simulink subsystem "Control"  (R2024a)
settings: Solver=VariableStepAuto  StartTime=0.0  StopTime=10.0  RelTol=1e-3
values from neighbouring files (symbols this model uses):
  Control = ControlType.Simple    [TotemPole_PFCData.m]
  Tsc_fast = 1e-5    (= 1e-05)    [TotemPole_PFCData.m]
  Tsc_slow = 0.01    [TotemPole_PFCData.m]
undefined symbols (not defined in the file or in its folder): I
libraries: simulink x10, simulink_extras x2, slpidlib x2, dspsigops x1

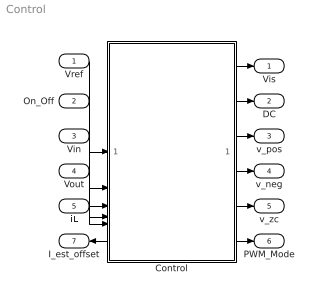
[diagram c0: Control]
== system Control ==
  Vref : Inport
  On_Off : Inport  Port=2
  Vin : Inport  Port=3
  Vout : Inport  Port=4
  iL : Inport  Port=5
  Control : Subsystem  Variant=on  VariantControl=Control
  Vis : Outport
  DC : Outport  Port=2
  v_pos : Outport  Port=3
  v_neg : Outport  Port=4
  v_zc : Outport  Port=5
  PWM_Mode : Outport  Port=6
  I_est_offset : Outport  Port=7
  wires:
  On_Off/1 -> Control/2(On_Off)
  iL/1 -> Control/5(iL)
  Control/6(PWM_Mode) -> PWM_Mode/1
  Vin/1 -> Control/3(Vin)
  Vout/1 -> Control/4(Vout)
  Control/1(Vis) -> Vis/1
  Control/2(DC) -> DC/1
  Control/3(v_pos) -> v_pos/1
  Control/4(v_neg) -> v_neg/1
  Control/5(v_zc) -> v_zc/1
  Control/7(I_est_offset) -> I_est_offset/1
  Vref/1 -> Control/1(Vref)

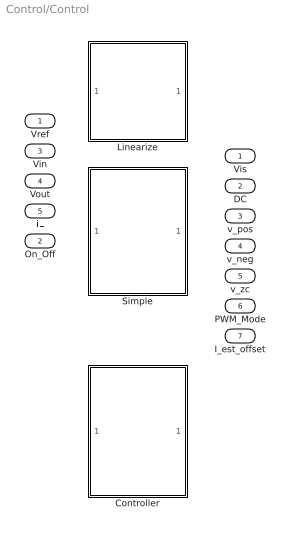
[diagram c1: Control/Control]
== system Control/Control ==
  Vref : Inport
  On_Off : Inport  Port=2
  Vin : Inport  Port=3
  Vout : Inport  Port=4
  iL : Inport  Port=5
  Controller : Subsystem  VariantControl=Control == ControlType.Detailed
  Linearize : Subsystem  VariantControl=Control == ControlType.Linearization
  Simple : Subsystem  VariantControl=Control == ControlType.Simple
  Vis : Outport
  DC : Outport  Port=2
  v_pos : Outport  Port=3
  v_neg : Outport  Port=4
  v_zc : Outport  Port=5
  PWM_Mode : Outport  Port=6
  I_est_offset : Outport  Port=7

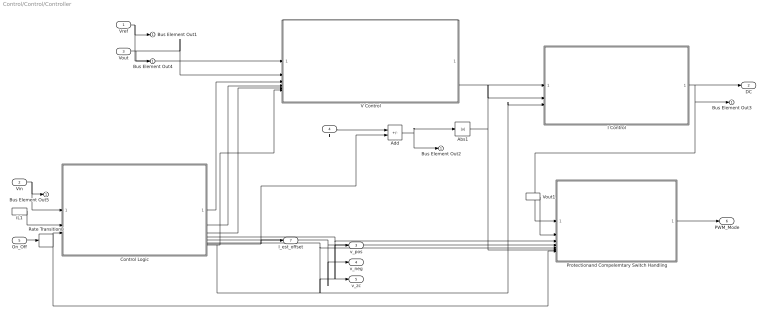
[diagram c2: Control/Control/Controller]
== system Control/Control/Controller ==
  Vref : Inport
  Vin : Inport  Port=2
  Vout : Inport  Port=3
  iL : Inport  Port=4
  On_Off : Inport  Port=5
  Abs1 : Abs
  Add : Sum  Inputs=+-
  Control Logic : Subsystem
  I Control : ModelReference  ModelNameDialog=I_Control  ModelReferenceVersion=9.283  CopyOfModelProtected=on
  Protectionand Compelemtary Switch Handling : Subsystem
  Rate Transition8 : RateTransition  OutPortSampleTime=1/100e3
  V Control : Subsystem
  Vout1 : InportShadow  Port=3
  iL1 : InportShadow  Port=4
  Bus Element Out{1..5} (5 alike) : Outport
  DC : Outport  Port=2
  v_pos : Outport  Port=3
  v_neg : Outport  Port=4
  v_zc : Outport  Port=5
  PWM_Mode : Outport  Port=6
  I_est_offset : Outport  Port=7
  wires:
  Add/1 -> Abs1/1, Bus Element Out2/1
  iL/1 -> Add/1
  Vref/1 -> Bus Element Out1/1, V Control/1(Vref)
  I Control/1 -> Protectionand Compelemtary Switch Handling/1(DC), Bus Element Out3/1, DC/1
  V Control/1(I_slowref) -> I Control/1
  Vin/1 -> Bus Element Out5/1, Control Logic/1(Vin)
  iL1/1 -> Control Logic/2(Iin)
  On_Off/1 -> Rate Transition8/1
  Control Logic/1(Vin_scaled) -> V Control/3(Vin_scaled)
  Control Logic/2(redge) -> V Control/4(redge)
  Control Logic/3(fedge) -> V Control/5(fedge)
  Control Logic/7(I_est_offset) -> I_est_offset/1, Add/2
  Vout/1 -> Bus Element Out4/1, V Control/2(Vout)
  Control Logic/6(V_zc) -> v_zc/1, Protectionand Compelemtary Switch Handling/5(vin_zc)
  Control Logic/4(V_pos) -> Protectionand Compelemtary Switch Handling/3(vin_p), v_pos/1
  Control Logic/5(V_neg) -> v_neg/1, Protectionand Compelemtary Switch Handling/4(vin_n)
  Abs1/1 -> Protectionand Compelemtary Switch Handling/6(I_abs), I Control/2
  Protectionand Compelemtary Switch Handling/1(PWM_Mode) -> PWM_Mode/1
  Vout1/1 -> Protectionand Compelemtary Switch Handling/2(Vout)
  Control Logic/8(EN_ALIGN) -> I Control/3, V Control/6(On_Off1)
  Rate Transition8/1 -> Protectionand Compelemtary Switch Handling/7(On_off_1), Control Logic/3(EN_M)

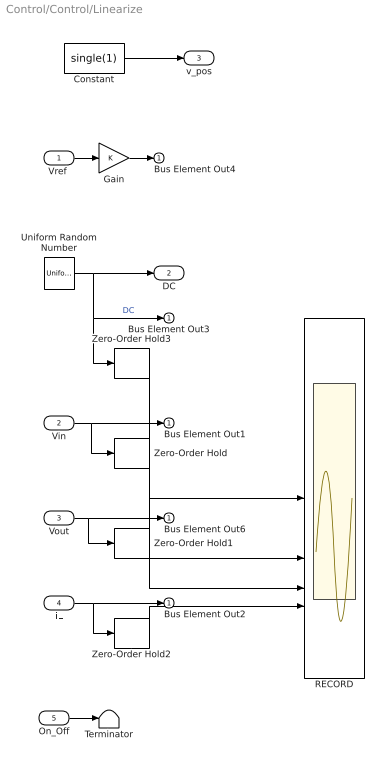
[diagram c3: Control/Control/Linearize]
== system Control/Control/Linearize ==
  "Vref " : Inport
  Vin : Inport  Port=2
  Vout : Inport  Port=3
  iL : Inport  Port=4
  On_Off : Inport  Port=5
  Constant : Constant  Value=single(1)
  Gain : Gain
  RECORD : Scope  NumInputPorts=4
  Terminator : Terminator
  Uniform Random Number : UniformRandomNumber  Minimum=-0.1  Maximum=0.1  SampleTime=Tsc_fast
  Zero-Order Hold{,1..3} (4 alike) : ZeroOrderHold  SampleTime=Tsc_fast
  Bus Element Out{1..4,6} (5 alike) : Outport
  DC : Outport  Port=2
  v_pos : Outport  Port=3
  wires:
  iL/1 -> Zero-Order Hold2/1, Bus Element Out2/1
  Vout/1 -> Zero-Order Hold1/1, Bus Element Out6/1
  Vin/1 -> Zero-Order Hold/1, Bus Element Out1/1
  Uniform Random Number/1 -> Bus Element Out3/1, Zero-Order Hold3/1, DC/1  "DC"
  Constant/1 -> v_pos/1
  Zero-Order Hold3/1 -> RECORD/1
  Zero-Order Hold/1 -> RECORD/2
  Zero-Order Hold1/1 -> RECORD/3
  Zero-Order Hold2/1 -> RECORD/4
  "Vref "/1 -> Gain/1
  Gain/1 -> Bus Element Out4/1
  On_Off/1 -> Terminator/1

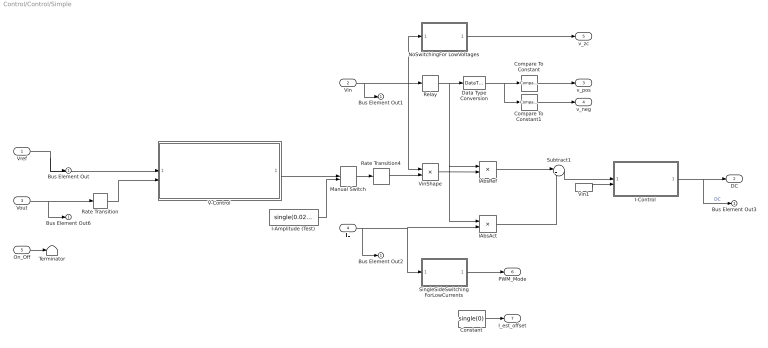
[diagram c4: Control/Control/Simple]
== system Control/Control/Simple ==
  Vref : Inport
  Vin : Inport  Port=2
  Vout : Inport  Port=3
  iL : Inport  Port=4
  On_Off : Inport  Port=5
  Compare To Constant : simulink/Logic and Bit Operations/Compare To Constant  relop===  const=1  OutDataTypeStr=boolean
  Compare To Constant1 : simulink/Logic and Bit Operations/Compare To Constant  relop===  const=-1  OutDataTypeStr=boolean
  Constant : Constant  Value=single(0)  SampleTime=Tsc_fast
  Data Type Conversion : DataTypeConversion  OutDataTypeStr=int8
  I-Amplitude (Test) : Constant  Value=single(0.025*10)  SampleTime=Tsc_fast
  I-Control : Subsystem  Variant=on  VariantControl=I-Control
  IAbsAct : Product
  IAbsRef : Product
  Manual Switch : ManualSwitch
  NoSwitchingFor LowVoltages : Subsystem  mask{vTh=2, perc=4}
      mask prompts: vTh "Voltage Threshold [V]"; perc "Hysteresis [+/- %]"
  Rate Transition : RateTransition  OutPortSampleTime=Tsc_slow
  Rate Transition4 : RateTransition  Deterministic=off  OutPortSampleTime=Tsc_fast
  Relay : Relay  OnSwitchValue=0.08  OffSwitchValue=-0.08  OffOutputValue=-1  ZeroCross=off
  SingleSideSwitching ForLowCurrents : Subsystem  mask{iTh=2, hyst=0.1}
      mask prompts: iTh "Current Threshold [A]"; hyst "Hysteresis [+/- A]"
  Subtract1 : Sum  Inputs=|+-
  Terminator : Terminator
  V-Control : Subsystem
  Vin1 : InportShadow  Port=2
  VinShape : Product
  Bus Element Out{,1..3,6} (5 alike) : Outport
  DC : Outport  Port=2
  v_pos : Outport  Port=3
  v_neg : Outport  Port=4
  v_zc : Outport  Port=5
  PWM_Mode : Outport  Port=6
  I_est_offset : Outport  Port=7
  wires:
  Rate Transition/1 -> V-Control/2(V_out)
  I-Control/1(DC) -> DC/1, Bus Element Out3/1  "DC"
  Vin1/1 -> I-Control/2(Vin)
  IAbsRef/1 -> Subtract1/1
  IAbsAct/1 -> Subtract1/2
  Constant/1 -> I_est_offset/1
  Vin/1 -> Relay/1, NoSwitchingFor LowVoltages/1(v), VinShape/1, Bus Element Out1/1
  VinShape/1 -> IAbsRef/2
  Rate Transition4/1 -> VinShape/2
  Vout/1 -> Rate Transition/1, Bus Element Out6/1
  I-Amplitude (Test)/1 -> Manual Switch/2
  Vref/1 -> Bus Element Out/1, V-Control/1(V_ref)
  SingleSideSwitching ForLowCurrents/1(PWM_Mode) -> PWM_Mode/1
  NoSwitchingFor LowVoltages/1(v_zc) -> v_zc/1
  Relay/1 -> Data Type Conversion/1, IAbsAct/1, IAbsRef/1
  Data Type Conversion/1 -> Compare To Constant1/1, Compare To Constant/1
  Subtract1/1 -> I-Control/1(delta_I)
  V-Control/1("I_ref ") -> Manual Switch/1
  Manual Switch/1 -> Rate Transition4/1
  iL/1 -> IAbsAct/2, SingleSideSwitching ForLowCurrents/1(i), Bus Element Out2/1
  On_Off/1 -> Terminator/1
  Compare To Constant/1 -> v_pos/1
  Compare To Constant1/1 -> v_neg/1

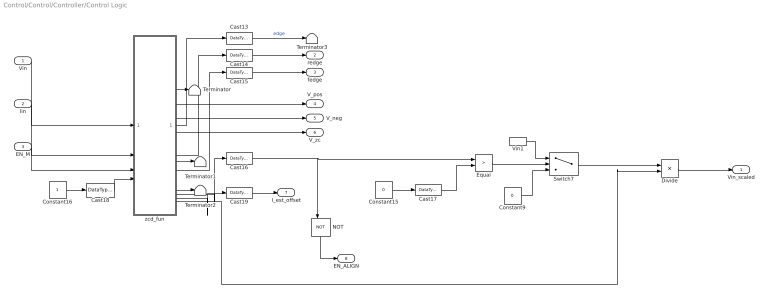
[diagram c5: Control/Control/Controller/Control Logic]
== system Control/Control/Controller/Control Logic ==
  Vin : Inport
  Iin : Inport  Port=2
  EN_M : Inport  Port=3
  Cast{13..17} (5 alike) : DataTypeConversion  OutDataTypeStr=boolean
  Cast18 : DataTypeConversion  OutDataTypeStr=single
  Cast19 : DataTypeConversion  OutDataTypeStr=single
  Constant15 : Constant  Value=0  OutDataTypeStr=single
  Constant16 : Constant
  Constant9 : Constant  Value=0  OutDataTypeStr=single
  Divide : Product  Inputs=**
  Equal : RelationalOperator  Operator=>  OutDataTypeStr=boolean  RndMeth=Simplest
  NOT : Logic  Operator=NOT  IconShape=distinctive  AllPortsSameDT=off  OutDataTypeStr=boolean
  Switch7 : Switch  Criteria=u2 > Threshold
  Terminator{,1..3} (4 alike) : Terminator
  Vin1 : InportShadow
  zcd_fun : MATLAB Function  TreatAsAtomicUnit=on
  Vin_scaled : Outport
  redge : Outport  Port=2
  fedge : Outport  Port=3
  V_pos : Outport  Port=4
  V_neg : Outport  Port=5
  V_zc : Outport  Port=6
  I_est_offset : Outport  Port=7
  EN_ALIGN : Outport  Port=8
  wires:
  zcd_fun/12(Vrms_inv2_o) -> Divide/2
  EN_M/1 -> zcd_fun/3(EN_M_in)
  Cast14/1 -> redge/1
  Constant9/1 -> Switch7/3
  Cast16/1 -> Equal/1, NOT/1
  Vin1/1 -> Switch7/1
  zcd_fun/5(V_pos) -> V_pos/1
  Iin/1 -> zcd_fun/2(Iin)
  Cast18/1 -> zcd_fun/4(Vth_in)
  zcd_fun/11(cedge) -> Terminator2/1
  Vin/1 -> zcd_fun/1(Vin)
  zcd_fun/3(fedge) -> Cast15/1
  zcd_fun/1(edge) -> Cast13/1
  Constant16/1 -> Cast18/1
  Equal/1 -> Switch7/2
  zcd_fun/2(redge) -> Cast14/1
  Cast19/1 -> I_est_offset/1
  Cast15/1 -> fedge/1
  zcd_fun/8(En_pos_align) -> Cast16/1
  Switch7/1 -> Divide/1
  Constant15/1 -> Cast17/1
  zcd_fun/10(I_offset2_o) -> Cast19/1
  Cast17/1 -> Equal/2
  Cast13/1 -> Terminator3/1  "edge"
  zcd_fun/4(Vpeak_o) -> Terminator/1
  zcd_fun/9(I_offset_o) -> Terminator1/1
  zcd_fun/7(V_zc) -> V_zc/1
  zcd_fun/6(V_neg) -> V_neg/1
  Divide/1 -> Vin_scaled/1
  NOT/1 -> EN_ALIGN/1

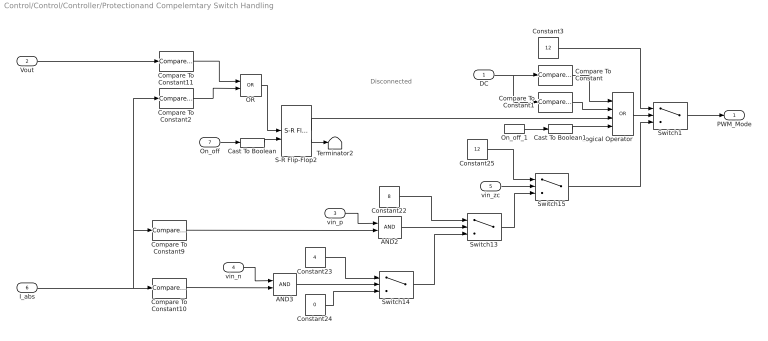
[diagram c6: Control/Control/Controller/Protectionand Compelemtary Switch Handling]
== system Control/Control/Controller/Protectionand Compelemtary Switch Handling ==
  note: Disconnected
  DC : Inport
  Vout : Inport  Port=2
  vin_p : Inport  Port=3
  vin_n : Inport  Port=4
  vin_zc : Inport  Port=5
  I_abs : Inport  Port=6
  On_off : Inport  Port=7
  AND2 : Logic  IconShape=distinctive  AllPortsSameDT=off  OutDataTypeStr=boolean
  AND3 : Logic  IconShape=distinctive  AllPortsSameDT=off  OutDataTypeStr=boolean
  Cast To Boolean : DataTypeConversion  OutDataTypeStr=boolean
  Cast To Boolean1 : DataTypeConversion  OutDataTypeStr=boolean
  Compare To Constant : simulink/Logic and Bit Operations/Compare To Constant  relop=<=  const=-0.001  OutDataTypeStr=boolean
  Compare To Constant1 : simulink/Logic and Bit Operations/Compare To Constant  relop=>=  const=1.1  OutDataTypeStr=boolean
  Compare To Constant10 : simulink/Logic and Bit Operations/Compare To Constant  relop=<  const=2  OutDataTypeStr=boolean
  Compare To Constant11 : simulink/Logic and Bit Operations/Compare To Constant  relop=>=  const=80  OutDataTypeStr=boolean
  Compare To Constant2 : simulink/Logic and Bit Operations/Compare To Constant  relop=>=  const=25  OutDataTypeStr=boolean
  Compare To Constant9 : simulink/Logic and Bit Operations/Compare To Constant  relop=<  const=2  OutDataTypeStr=boolean
  Constant22 : Constant  Value=8  OutDataTypeStr=uint16
  Constant23 : Constant  Value=4  OutDataTypeStr=uint16
  Constant24 : Constant  Value=0  OutDataTypeStr=uint16
  Constant25 : Constant  Value=12  OutDataTypeStr=uint16
  Constant3 : Constant  Value=12  OutDataTypeStr=uint16
  Logical Operator : Logic  Operator=OR  Inputs=4  AllPortsSameDT=off  OutDataTypeStr=boolean
  OR : Logic  Operator=OR  IconShape=distinctive  AllPortsSameDT=off  OutDataTypeStr=boolean
  On_off_1 : InportShadow  Port=7
  S-R Flip-Flop2 : simulink_extras/Flip Flops/S-R Flip-Flop  initial_condition=0
  Switch{1,13..15} (4 alike) : Switch  Criteria=u2 > Threshold
  Terminator2 : Terminator
  PWM_Mode : Outport
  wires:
  Compare To Constant10/1 -> AND3/2
  Switch1/1 -> PWM_Mode/1
  S-R Flip-Flop2/2 -> Terminator2/1
  Constant25/1 -> Switch15/1
  AND3/1 -> Switch14/2
  Switch15/1 -> Switch1/3
  Cast To Boolean/1 -> S-R Flip-Flop2/2
  OR/1 -> S-R Flip-Flop2/1
  Constant3/1 -> Switch1/1
  vin_zc/1 -> Switch15/2
  Constant24/1 -> Switch14/3
  Compare To Constant9/1 -> AND2/2
  vin_p/1 -> AND2/1
  Logical Operator/1 -> Switch1/2
  Compare To Constant11/1 -> OR/1
  Switch13/1 -> Switch15/3
  Compare To Constant/1 -> Logical Operator/1
  DC/1 -> Compare To Constant/1, Compare To Constant1/1
  Compare To Constant1/1 -> Logical Operator/2
  AND2/1 -> Switch13/2
  Constant22/1 -> Switch13/1
  Switch14/1 -> Switch13/3
  vin_n/1 -> AND3/1
  Vout/1 -> Compare To Constant11/1
  Constant23/1 -> Switch14/1
  On_off/1 -> Cast To Boolean/1
  I_abs/1 -> Compare To Constant2/1, Compare To Constant9/1, Compare To Constant10/1
  S-R Flip-Flop2/1 -> Logical Operator/3
  On_off_1/1 -> Cast To Boolean1/1
  Compare To Constant2/1 -> OR/2
  Cast To Boolean1/1 -> Logical Operator/4

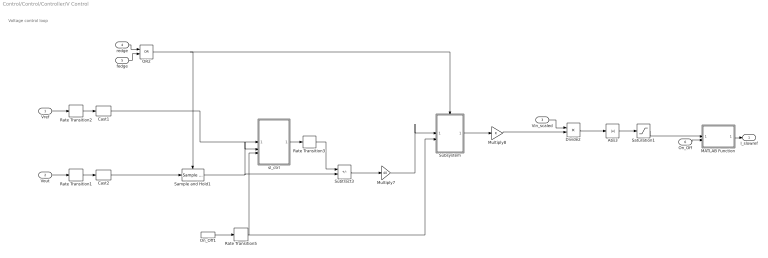
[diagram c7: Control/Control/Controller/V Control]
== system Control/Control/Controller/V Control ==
  note: Voltage control loop
  Vref : Inport
  Vout : Inport  Port=2
  Vin_scaled : Inport  Port=3
  redge : Inport  Port=4
  fedge : Inport  Port=5
  On_Off : Inport  Port=6
  Abs3 : Abs
  Cast1 : DataTypeConversion  OutDataTypeStr=single
  Cast2 : DataTypeConversion  OutDataTypeStr=single
  Divide2 : Product  Inputs=**
  MATLAB Function : MATLAB Function  TreatAsAtomicUnit=on
  Multiply7 : Gain  Gain=40
  Multiply8 : Gain
  OR2 : Logic  Operator=OR  IconShape=distinctive  AllPortsSameDT=off  OutDataTypeStr=boolean
  On_Off1 : InportShadow  Port=6
  Rate Transition1 : RateTransition  OutPortSampleTime=Tsc_fast
  Rate Transition2 : RateTransition  OutPortSampleTime=Tsc_slow
  Rate Transition3 : RateTransition  OutPortSampleTime=Tsc_slow
  Rate Transition5 : RateTransition  OutPortSampleTime=Tsc_slow
  Sample and Hold1 : dspsigops/Sample and Hold  trig=Rising edge  initCond=0  latchinput=off
  Saturation1 : Saturate  UpperLimit=30  LowerLimit=-30
  Subsystem : Subsystem
  Subtract3 : Sum  Inputs=+-
  sl_ctrl : MATLAB Function  TreatAsAtomicUnit=on
  I_slowref : Outport
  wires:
  Rate Transition5/1 -> Subsystem/2(In2), sl_ctrl/3(RST)
  Saturation1/1 -> MATLAB Function/1(I_ref)
  Rate Transition1/1 -> Cast2/1
  Rate Transition3/1 -> Subtract3/1
  OR2/1 -> Sample and Hold1/Trigger, Subsystem/Enable
  Abs3/1 -> Saturation1/1
  Cast1/1 -> sl_ctrl/1(V_ref)
  Vin_scaled/1 -> Divide2/1
  sl_ctrl/1(V_slowref) -> Rate Transition3/1
  Rate Transition2/1 -> Cast1/1
  Vout/1 -> Rate Transition1/1
  redge/1 -> OR2/1
  Subtract3/1 -> Multiply7/1
  Sample and Hold1/1 -> Subtract3/2, sl_ctrl/2(V_init)
  Multiply7/1 -> Subsystem/1(In1)
  Subsystem/1(Out1) -> Multiply8/1
  fedge/1 -> OR2/2
  Cast2/1 -> Sample and Hold1/1
  Divide2/1 -> Abs3/1
  MATLAB Function/1(I_slowref) -> I_slowref/1
  Multiply8/1 -> Divide2/2
  On_Off/1 -> MATLAB Function/2(RST)
  Vref/1 -> Rate Transition2/1
  On_Off1/1 -> Rate Transition5/1

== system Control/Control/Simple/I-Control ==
  delta_I : Inport
  Vin : Inport  Port=2
  IIR_Control : Subsystem  VariantControl=IControl == IControlType.IIR_2p2z
  PI Controller : Subsystem  VariantControl=IControl == IControlType.PI
  DC : Outport

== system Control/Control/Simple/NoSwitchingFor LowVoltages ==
  v : Inport
  Abs : Abs  ZeroCross=off
  NOT : Logic  Operator=NOT  IconShape=distinctive  AllPortsSameDT=off  OutDataTypeStr=boolean
  Relay : Relay  OnSwitchValue=vTh*(1+perc/100)  OffSwitchValue=vTh*(1-perc/100)  OutDataTypeStr=boolean  ZeroCross=off
  v_zc : Outport
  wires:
  Abs/1 -> Relay/1
  v/1 -> Abs/1
  Relay/1 -> NOT/1
  NOT/1 -> v_zc/1

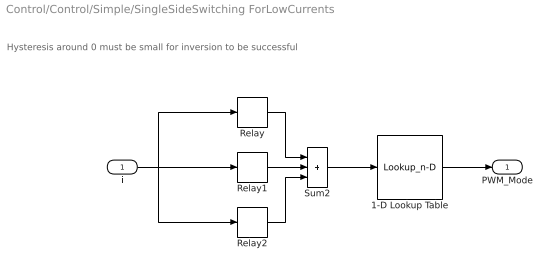
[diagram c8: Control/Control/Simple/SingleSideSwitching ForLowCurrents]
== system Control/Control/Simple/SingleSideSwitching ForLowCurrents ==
  note: Hysteresis around 0 must be small for inversion to be successful
  i : Inport
  1-D Lookup Table : Lookup_n-D  NumberOfTableDimensions=1  LookupTableObject=''  BreakpointsForDimension1=[0,1,2,3]  BreakpointsForDimension1FirstPoint=10  BreakpointsForDimension2FirstPoint=10  BreakpointsForDimension1Spacing=12  BreakpointsForDimension2Spacing=12  IndexSearchMethod=Evenly spaced points  Table=[0,4,8,0]  InterpMethod=Flat  DiagnosticForOutOfRangeInput=Error  InternalRulePriority=Speed  RndMeth=Simplest
  Relay : Relay  OnSwitchValue=iTh+hyst  OffSwitchValue=iTh-hyst  OutDataTypeStr=int8  ZeroCross=off
  Relay1 : Relay  OnSwitchValue=0.02  OffSwitchValue=-0.02  OutDataTypeStr=int8  ZeroCross=off
  Relay2 : Relay  OnSwitchValue=-iTh+hyst  OffSwitchValue=-iTh-hyst  OutDataTypeStr=int8  ZeroCross=off
  Sum2 : Sum  Inputs=+++
  PWM_Mode : Outport
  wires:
  Relay1/1 -> Sum2/2
  i/1 -> Relay2/1, Relay1/1, Relay/1
  Relay2/1 -> Sum2/3
  Relay/1 -> Sum2/1
  Sum2/1 -> 1-D Lookup Table/1
  1-D Lookup Table/1 -> PWM_Mode/1

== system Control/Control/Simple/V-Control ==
  V_ref : Inport
  V_out : Inport  Port=2
  "PI Controller no Saturation " : slpidlib/PID Controller  Controller=PI  Form=Parallel  TimeDomain=Discrete-time  UseExternalTs=off  SampleTime=Tsc_slow  IntegratorMethod=Forward Euler  FilterMethod=Forward Euler  ControllerParametersSource=internal  P=0.08  I=0.7  UseKiTs=off  D=0  UseExternalDerivativeSource=off  N=100  UseFilter=on  TunerSelectOption=Transfer Function Based (PID Tuner App)  ZeroCross=off  InitialConditionSource=internal  InitialConditionForIntegrator=0  InitialConditionForFilter=0  DifferentiatorICPrevScaledInput=0  ExternalReset=none  TrackingMode=off  Kt=1  LimitOutput=on  SatLimitsSource=internal  UpperSaturationLimit=0.5  LowerSaturationLimit=-1  LinearizeAsGain=on  AntiWindupMode=clamping  Kb=1  LimitIntegrator=off  UpperIntegratorSaturationLimit=inf  LowerIntegratorSaturationLimit=-inf  POutMin=[]  POutMax=[]  IOutMin=[]  IOutMax=[]  DOutMin=[]  DOutMax=[]  NOutMin=[]  NOutMax=[]  SumOutMin=[]  SumOutMax=[]  SaturationOutMin=[]  SaturationOutMax=[]  PParamMin=[]  PParamMax=[]  IParamMin=[]  IParamMax=[]  DParamMin=[]  DParamMax=[]  NParamMin=[]  NParamMax=[]  KbParamMin=[]  KbParamMax=[]  KtParamMin=[]  KtParamMax=[]  KbOutMin=[]  KbOutMax=[]  KtOutMin=[]  KtOutMax=[]  IntegratorOutMin=[]  IntegratorOutMax=[]  FilterOutMin=[]  FilterOutMax=[]  SumI1OutMin=[]  SumI1OutMax=[]  SumI2OutMin=[]  SumI2OutMax=[]  SumI3OutMin=[]  SumI3OutMax=[]  SumI4OutMin=[]  SumI4OutMax=[]  SumDOutMin=[]  SumDOutMax=[]  DifferentiatorOutMin=[]  DifferentiatorOutMax=[]  FilterDiffOutCoefMin=[]  FilterDiffOutCoefMax=[]  ReciprocalOutMin=[]  ReciprocalOutMax=[]  SumDenOutMin=[]  SumDenOutMax=[]  SumNumOutMin=[]  SumNumOutMax=[]  DivideOutMin=[]  DivideOutMax=[]  UdiffTsProdOutMin=[]  UdiffTsProdOutMax=[]  NTsProdOutMin=[]  NTsProdOutMax=[]  UintegralTsProdOutMin=[]  UintegralTsProdOutMax=[]  UngainTsProdOutMin=[]  UngainTsProdOutMax=[]  ClampingZeroOutDataTypeStr=Inherit: Inherit via back propagation  ClampingZeroOutMin=[]  ClampingZeroOutMax=[]  FilterDenConstantOutDataTypeStr=Inherit: Inherit via back propagation  FilterDenConstantOutMin=[]  FilterDenConstantOutMax=[]  PCopyOutDataTypeStr=Inherit: Inherit via back propagation  PCopyOutMin=[]  PCopyOutMax=[]  NCopyOutDataTypeStr=Inherit: Inherit via back propagation  NCopyOutMin=[]  NCopyOutMax=[]  IntegratorContinuousStateAttributes=''  IntegratorStateMustResolveToSignalObject=off  IntegratorRTWStateStorageClass=Auto  FilterContinuousStateAttributes=''  FilterStateMustResolveToSignalObject=off  FilterRTWStateStorageClass=Auto  ParallelPVariant=InternalParameters  IdealPVariant=Disabled  IVariant=InternalParameters  DVariant=Disabled  IntegratorVariant=Discrete  SatVariant=Enabled  AWVariant=DiscClampingParallel  PCopyVariant=Disabled  TRVariant=Disabled  FdbkBlocksVariant=Forward  IdealPFdbkVariant=Disabled  SatFdbkVariant=Disabled  DerivativeFilterVariant=Disabled  NVariant=Disabled  NCopyVariant=Disabled_SignalSpec  FilterICVariant=Disabled  IntegratorICVariant=InternalICs  ExternalResetVariant=Disabled  TRSumVariant=Passthrough  SumFdbkVariant=Disabled  SumVariant=Sum_PI  TsampFilterVariant=InternalTs  TsampNgainVariant=Passthrough  TsampIntegralVariant=Disabled_SignalSpec  ExternalSaturationOutDataTypeStr=Inherit: Same as second input  DerivativeSourceVariant=Disabled
  Sum : Sum  Inputs=|+-
  "I_ref " : Outport
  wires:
  Sum/1 -> "PI Controller no Saturation "/1
  V_ref/1 -> Sum/1
  V_out/1 -> Sum/2
  "PI Controller no Saturation "/1 -> "I_ref "/1  "DC"

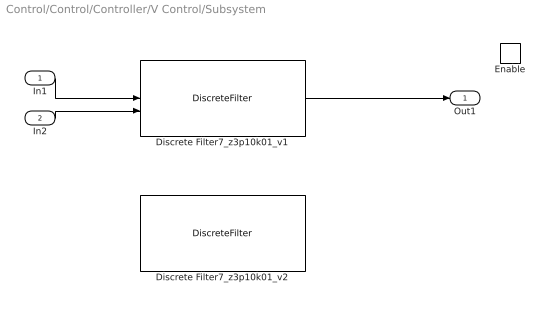
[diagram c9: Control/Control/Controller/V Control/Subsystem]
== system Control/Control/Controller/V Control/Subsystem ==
  In1 : Inport
  In2 : Inport  Port=2
  Enable : EnablePort
  Discrete Filter7_z3p10k01_v1 : DiscreteFilter  Numerator=[0.159 0.030 -0.130]  Denominator=[1 -0.120 -0.880]  InputProcessing=Columns as channels (frame based)  ExternalReset=Either  FilterStructure=Direct form II transposed  a0EqualsOne=on
  Discrete Filter7_z3p10k01_v2 : DiscreteFilter  Commented=on  Numerator=[3.188 0.591 -2.597]  Denominator=[1 -0.120 -0.880]  InputProcessing=Columns as channels (frame based)  ExternalReset=Either  FilterStructure=Direct form II transposed  a0EqualsOne=on
  Out1 : Outport
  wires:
  In2/1 -> Discrete Filter7_z3p10k01_v1/2
  Discrete Filter7_z3p10k01_v1/1 -> Out1/1
  In1/1 -> Discrete Filter7_z3p10k01_v1/1

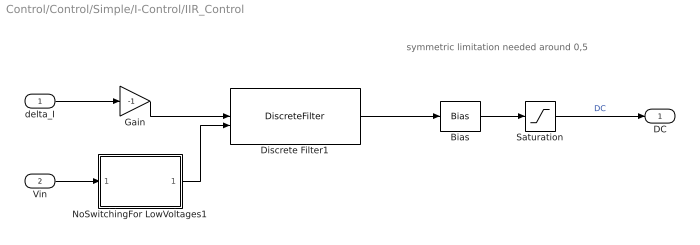
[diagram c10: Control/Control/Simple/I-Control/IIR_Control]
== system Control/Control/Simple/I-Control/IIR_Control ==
  note: symmetric limitation needed around 0,5
  delta_I : Inport
  Vin : Inport  Port=2
  Bias : Bias  Commented=through  Bias=1
  Discrete Filter1 : DiscreteFilter  Numerator=[0.073 0.003 -0.070]  Denominator=[1 -0.778 -0.222]  ExternalReset=Either  FilterStructure=Direct form II transposed  a0EqualsOne=on
  Gain : Gain  Gain=-1
  NoSwitchingFor LowVoltages1 : Subsystem  mask{vTh=2}
      mask prompts: vTh "Voltage Threshold [V]"
  Saturation : Saturate  UpperLimit=0.98  LowerLimit=0.02
  DC : Outport
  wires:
  Gain/1 -> Discrete Filter1/1
  Bias/1 -> Saturation/1
  delta_I/1 -> Gain/1
  Discrete Filter1/1 -> Bias/1
  Saturation/1 -> DC/1  "DC"
  Vin/1 -> NoSwitchingFor LowVoltages1/1(v)
  NoSwitchingFor LowVoltages1/1(Reset) -> Discrete Filter1/2

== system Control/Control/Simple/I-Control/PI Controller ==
  delta_I : Inport
  PI Controller Saturation for DC = 0.02..0.98 Anti-windup : slpidlib/PID Controller  Controller=PI  Form=Parallel  TimeDomain=Discrete-time  UseExternalTs=off  SampleTime=Tsc_fast  IntegratorMethod=Forward Euler  FilterMethod=Forward Euler  ControllerParametersSource=internal  P=0.25  I=4000  UseKiTs=off  D=0  UseExternalDerivativeSource=off  N=100  UseFilter=on  TunerSelectOption=Transfer Function Based (PID Tuner App)  ZeroCross=off  InitialConditionSource=internal  InitialConditionForIntegrator=0.02  InitialConditionForFilter=0  DifferentiatorICPrevScaledInput=0  ExternalReset=none  TrackingMode=off  Kt=1  LimitOutput=on  SatLimitsSource=internal  UpperSaturationLimit=0.98  LowerSaturationLimit=0.02  LinearizeAsGain=on  AntiWindupMode=clamping  Kb=1  LimitIntegrator=off  UpperIntegratorSaturationLimit=inf  LowerIntegratorSaturationLimit=-inf  POutMin=[]  POutMax=[]  IOutMin=[]  IOutMax=[]  DOutMin=[]  DOutMax=[]  NOutMin=[]  NOutMax=[]  SumOutMin=[]  SumOutMax=[]  SaturationOutMin=[]  SaturationOutMax=[]  PParamMin=[]  PParamMax=[]  IParamMin=[]  IParamMax=[]  DParamMin=[]  DParamMax=[]  NParamMin=[]  NParamMax=[]  KbParamMin=[]  KbParamMax=[]  KtParamMin=[]  KtParamMax=[]  KbOutMin=[]  KbOutMax=[]  KtOutMin=[]  KtOutMax=[]  IntegratorOutMin=[]  IntegratorOutMax=[]  FilterOutMin=[]  FilterOutMax=[]  SumI1OutMin=[]  SumI1OutMax=[]  SumI2OutMin=[]  SumI2OutMax=[]  SumI3OutMin=[]  SumI3OutMax=[]  SumI4OutMin=[]  SumI4OutMax=[]  SumDOutMin=[]  SumDOutMax=[]  DifferentiatorOutMin=[]  DifferentiatorOutMax=[]  FilterDiffOutCoefMin=[]  FilterDiffOutCoefMax=[]  ReciprocalOutMin=[]  ReciprocalOutMax=[]  SumDenOutMin=[]  SumDenOutMax=[]  SumNumOutMin=[]  SumNumOutMax=[]  DivideOutMin=[]  DivideOutMax=[]  UdiffTsProdOutMin=[]  UdiffTsProdOutMax=[]  NTsProdOutMin=[]  NTsProdOutMax=[]  UintegralTsProdOutMin=[]  UintegralTsProdOutMax=[]  UngainTsProdOutMin=[]  UngainTsProdOutMax=[]  ClampingZeroOutDataTypeStr=Inherit: Inherit via back propagation  ClampingZeroOutMin=[]  ClampingZeroOutMax=[]  FilterDenConstantOutDataTypeStr=Inherit: Inherit via back propagation  FilterDenConstantOutMin=[]  FilterDenConstantOutMax=[]  PCopyOutDataTypeStr=Inherit: Inherit via back propagation  PCopyOutMin=[]  PCopyOutMax=[]  NCopyOutDataTypeStr=Inherit: Inherit via back propagation  NCopyOutMin=[]  NCopyOutMax=[]  IntegratorContinuousStateAttributes=''  IntegratorStateMustResolveToSignalObject=off  IntegratorRTWStateStorageClass=Auto  FilterContinuousStateAttributes=''  FilterStateMustResolveToSignalObject=off  FilterRTWStateStorageClass=Auto  ParallelPVariant=InternalParameters  IdealPVariant=Disabled  IVariant=InternalParameters  DVariant=Disabled  IntegratorVariant=Discrete  SatVariant=Enabled  AWVariant=DiscClampingParallel  PCopyVariant=Disabled  TRVariant=Disabled  FdbkBlocksVariant=Forward  IdealPFdbkVariant=Disabled  SatFdbkVariant=Disabled  DerivativeFilterVariant=Disabled  NVariant=Disabled  NCopyVariant=Disabled_SignalSpec  FilterICVariant=Disabled  IntegratorICVariant=InternalICs  ExternalResetVariant=Disabled  TRSumVariant=Passthrough  SumFdbkVariant=Disabled  SumVariant=Sum_PI  TsampFilterVariant=InternalTs  TsampNgainVariant=Passthrough  TsampIntegralVariant=Disabled_SignalSpec  ExternalSaturationOutDataTypeStr=Inherit: Same as second input  DerivativeSourceVariant=Disabled
  DC : Outport
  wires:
  PI Controller Saturation for DC = 0.02..0.98 Anti-windup/1 -> DC/1  "DC"
  delta_I/1 -> PI Controller Saturation for DC = 0.02..0.98 Anti-windup/1

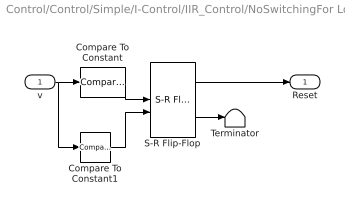
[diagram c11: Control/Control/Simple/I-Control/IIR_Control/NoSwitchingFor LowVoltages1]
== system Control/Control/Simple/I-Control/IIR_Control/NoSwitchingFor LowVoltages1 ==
  v : Inport
  Compare To Constant : simulink/Logic and Bit Operations/Compare To Constant  relop=>=  const=vTh  OutDataTypeStr=boolean  ZeroCross=off
  Compare To Constant1 : simulink/Logic and Bit Operations/Compare To Constant  relop=<=  const=-vTh  OutDataTypeStr=boolean  ZeroCross=off
  S-R Flip-Flop : simulink_extras/Flip Flops/S-R Flip-Flop  initial_condition=0
  Terminator : Terminator
  Reset : Outport
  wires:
  S-R Flip-Flop/1 -> Reset/1
  v/1 -> Compare To Constant1/1, Compare To Constant/1
  Compare To Constant/1 -> S-R Flip-Flop/1
  Compare To Constant1/1 -> S-R Flip-Flop/2
  S-R Flip-Flop/2 -> Terminator/1

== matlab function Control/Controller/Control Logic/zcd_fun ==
function [edge,redge,fedge, Vpeak_o, V_pos, V_neg, V_zc, En_pos_align, I_offset_o, I_offset2_o, cedge, Vrms_inv2_o] = zcd(Vin, Iin, EN_M_in,Vth_in)

persistent state;
persistent Vin_d1;
persistent Vdiff_d1;
persistent tmr;
persistent Vpeak;
persistent Vpeak_d1;
persistent En_pos_align_r;
persistent I_offset_r;
persistent I_offset_r2;
persistent Iin_d1;
persistent Cnt;
persistent Vrms;
persistent Vrms_d1;
persistent Accreg;
persistent Accreg_t;
persistent Cnt2;

S_POS = uint16(0);
S_NEG = uint16(1);
S_ZC = uint16(2);

VTH = single(Vth_in);
V_pos = uint16(0);
V_neg = uint16(0);
V_zc = uint16(0);

tmr_init = uint16(20);
edge = single(0);
redge = uint16(0);
nedge = uint16(0);
cedge = uint16(0);

En_pos_align = uint16(0);

off_update = uint16(0);

CUR_SCALE = 1/(25e-3/3.3*4096);
CNT_TH = uint32(500000);

CNT_TH2 = uint32(2000);

if isempty(state)
    state = S_ZC;
    Vin_d1 = single(0);
    tmr = uint16(tmr_init);
    Vpeak = single(0);
    Vpeak_d1 = single(0);
    En_pos_align_r = uint16(0);
    I_offset_r = single(-0.5);
    I_offset_r2 = single(-0.5);
    %Iin_d1 = single(2030);
    Iin_d1 = single(0);
    Cnt = uint32(0);
    Vrms = single(23.0);
    Vrms_d1 = single(23.0);
    Accreg = single(0.0);
    Accreg_t = single(0.0);
    Cnt2 = uint32(0);
end

Vdiff = Vin - Vin_d1;

if ((Vin > VTH) && (Vin_d1 <= VTH) ) 
    edge = single(-1);
    redge = uint16(1);
    fedge = uint16(0);
elseif ((Vin <= -VTH) && (Vin_d1 > -VTH) )
    edge = single(1);
    redge = uint16(0);
    fedge = uint16(1);
else
    edge = single(0);
    redge = uint16(0);
    fedge = uint16(0);
end

if (redge)
    Vpeak_d1 = Vpeak;
end

if (redge)
   Vpeak = single(0);
else
  if (Vin > Vpeak)
      Vpeak = Vin;
  end
end


if (Vin > VTH) 
    V_pos = uint16(1);
    V_neg = uint16(0);
    V_zc = uint16(0);
    tmr = tmr_init;
elseif (Vin <= -VTH)
    V_pos = uint16(0);
    V_neg = uint16(1);
    V_zc = uint16(0);
else
    V_pos = uint16(0);
    V_neg = uint16(0);
    V_zc = uint16(1);
end

if (Cnt == CNT_TH)
    Cnt = uint32(0);
    off_update = uint16(1);
else
    Cnt = Cnt + uint32(1);
    off_update = uint16(0);
end

if ((Vin >= 0) && (Vin_d1 < 0)) 
    I_offset_r = single(Iin);
end

if (off_update)
    I_offset_r2 = I_offset_r;
end

I_offset_o = I_offset_r;
I_offset2_o = I_offset_r2;

if (EN_M_in > 0)
    En_pos_align_r = uint16(0);
elseif (redge)
    En_pos_align_r = uint16(1);
end

% if (redge)
%     En_pos_align_r = uint16(1);
% end

Rmsupd = uint32(0);

if (Cnt2 == CNT_TH2)
    Cnt2 = uint32(0);
    Accreg_t = Accreg + abs(Vin);
    Accreg_t = (Accreg / 2000) * single(1.1107207);
    Accreg = single(0.0);
    Rmsupd = uint32(1);
else
    Cnt2 = Cnt2 + uint32(1);
    Accreg = Accreg + abs(Vin);
    Accreg_t = single(0.0);
    Rrmsupd = uint32(0);
end

if (Rmsupd)
    Vrms = single(1.0) / (Accreg_t * Accreg_t);
end

Vrms_inv2_o = Vrms;

En_pos_align = En_pos_align_r;

Vin_d1 = Vin;
Vdiff_d1 = Vdiff;

Vpeak_o = Vpeak_d1;

y = edge;

Iin_d1 = Iin;

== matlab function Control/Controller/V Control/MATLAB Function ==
function I_slowref = CalcInc(I_ref, RST)

% persistent I_acc;
% 
% if isempty(I_acc)
%     I_acc = single(0.0);
% end
% 
% I_d = single(4/100e3);
% 
% if RST > 0
%     I_acc = single(0.0);
% elseif I_acc > I_ref
%     I_acc = I_acc - I_d;
% elseif I_acc < I_ref
%     I_acc = I_acc + I_d;
% else
%     I_acc = I_acc;
% end
% 
% I_slowref = I_acc;

I_slowref = single(0.0);

if RST > 0
    I_slowref = single(0.0);
else
    I_slowref = I_ref;
end

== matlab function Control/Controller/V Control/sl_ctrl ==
function V_slowref = CalcInc_V(V_ref, V_init, RST)

persistent V_acc;

if isempty(V_acc)
    V_acc = single(0.0);
end

V_d = single(4.0/100);

if RST > 0
    V_acc = V_init;
elseif V_acc > V_ref
    V_acc = V_acc - V_d;
elseif V_acc < V_ref
    V_acc = V_acc + V_d;
else
    V_acc = V_acc;
end

V_slowref = V_acc;

% 
% I_slowref = single(0.0);
% 
% if RST > 0
%     I_slowref = single(0.0);
% else
%     I_slowref = I_ref;
% end
